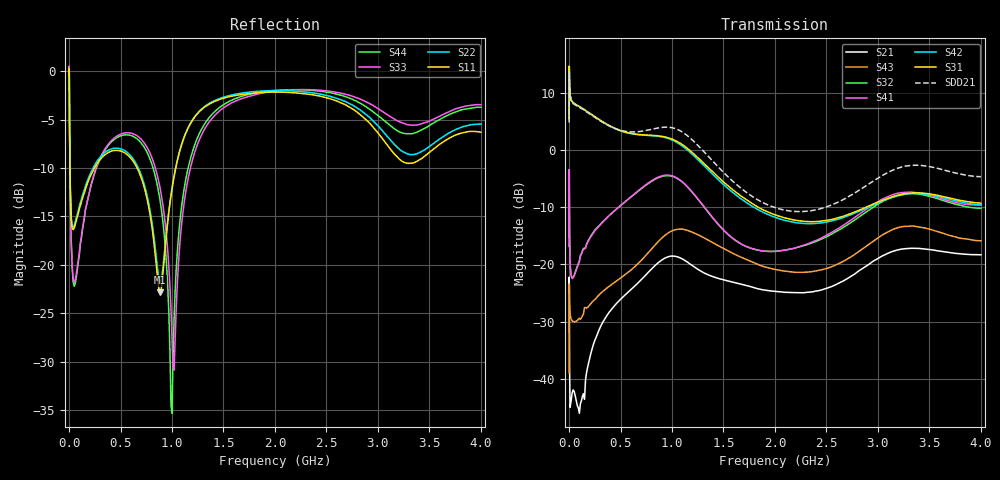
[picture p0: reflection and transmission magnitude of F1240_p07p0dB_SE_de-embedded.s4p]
! Integrated Device Technology
! Corporate Headquarters
! 6024 Silver Creek Valley Road
! San Jose, CA 95138  USA
! Phone:  1-408-284-8200
! Toll Free:  1-800-223-1366
! Webpage:  http://www.idt.com/
! Timing and RF Division
! 515 Groton Road, Suite 102
! Westford, MA 01886-6024
! Device:  F1240
! Description: Dual Intermediate Frequency Digital Variable Gain Amplifier
! Frequency:  10.0 -  500.00 MHz
! Package:  5x5 mm QFN Plastic Package: 32 pin
! Ports:  8 RF, 20 DC
!  Pin  1  = GA3 / Data  Pin 17  = RF OUT_B+
!  Pin  2  = GA4 / CLK  Pin 18  = RF OUT_B-
!  Pin  3  = GA5  Pin 19  = STBY_B
!  Pin  4  = VMODE  Pin 20  = Ground
!  Pin  5  = No Connect  Pin 21  = Ground
!  Pin  6  = GB5  Pin 22  = STB_A
!  Pin  7  = GB4  Pin 23  = RF OUT_A-  = Port 4
!  Pin  8  = GB3  Pin 24  = RF OUT_A+  = Port 3
!  Pin  9  = GB2  Pin 25  = GA0
!  Pin 10  = GB1  Pin 26  = ISET_A
!  Pin 11  = RF IN_B+  Pin 27  = VCC
!  Pin 12  = RF IN_B-  Pin 28  = Ground
!  Pin 13  = Ground  Pin 29  = RF IN_A-  = Port 2
!  Pin 14  = VCC  Pin 30  = RF IN_A+  = Port 1
!  Pin 15  = ISET_B  Pin 31  = GA1
!  Pin 16  = GB0  Pin 32  = GA2 / CSb
! Gain  = +19.5 dB
! State  = 1
! Voltage  = +5.00 V
! Current  = 85.292 mA (one channel only)
! Temperture  =  +25 C
! Test Date  =  2017-10-18
! Board  =  EB4031
! Data:  The device was measured on a custom evaluation board which has
!  individual transmission lines to the RF pins.  Data was collected
!  using a calibrated network analyzer.  The evaluation board was
!  de-embedded using Automatic Fixture Removal.
!  The reference plane is the edge of the package pin.
!  Only Channel A was measured.
!  This data is in single-ended operation.  If your needs are balanced
!  or differential S-parameters then this file needs to be used a
!  linear simulator.
! File Date:  2017-11-10  MJV
! Note:
!  Integrated Device Technology supplies this data as a sample of measured
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# Hz S dB R 100
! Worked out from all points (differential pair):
!   410 points, 500 kHz to 4 GHz, reference 100 ohm
!   strongest paths, dB at 500 kHz, 930 MHz, 1.96 GHz, 2.98 GHz, 4 GHz:
!     S31: 5.6, 2.4, -11.0, -9.2, -9.2
!     S42: 5.5, 2.2, -11.5, -9.4, -9.5
!     S41: -16.7, -4.4, -17.7, -9.2, -9.5
!     S32: -16.9, -4.5, -17.7, -9.7, -10.2
!     S43: -39.0, -14.9, -20.7, -15.6, -15.9
!     S21: -25.0, -18.9, -24.6, -19.2, -18.3
!   taken as a pair (ports 1,2 in; 3,4 out), SDD21 dB: 4.9, 4.1, -9.8, -5.1, -4.6
!   lowest |S11| = -22.8 dB at 880 MHz (marker M1), VSWR 1.16, Z = 111 + j10.7 ohm
!   |S11| at or under -10 dB: 8.743 MHz to 246.3 MHz (237.6 MHz wide, 186 % of centre); 661.2 MHz to 1.036 GHz (374.8 MHz wide, 44.2 % of centre)
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500000  -0.43 -5.5  -25.02 -6.0  -27.16 83.0  -57.48 70.7
        -25.00 -6.1  -0.43 -5.5  -57.70 72.0  -27.16 84.1
        5.57 -105.0  -16.87 -96.5  -0.51 1.5  -39.05 -86.1
        -16.72 -95.8  5.54 -103.9  -38.96 -85.7  -0.52 3.8
3000000  -2.38 -59.6  -27.90 -106.1  -15.26 28.3  -47.33 -69.5
         -27.98 -105.9  -2.34 -59.6  -47.16 -69.5  -15.27 28.4
         13.97 178.7  -7.17 153.0  -1.84 -54.9  -24.04 -164.6
         -7.26 152.8  13.97 178.9  -23.99 -164.6  -1.90 -54.7
3e7  -16.19 -116.0  -42.28 2.6  -15.36 -7.6  -48.21 102.3
     -42.48 1.7  -16.00 -116.1  -48.05 102.5  -15.34 -7.5
     8.53 162.3  -22.32 119.3  -20.05 -104.7  -30.02 162.9
     -22.48 119.8  8.56 162.4  -29.87 162.9  -20.34 -104.8
1.9e8  -11.26 -141.5  -37.59 56.7  -16.79 -48.0  -34.36 31.2
       -37.22 56.9  -10.99 -142.2  -34.33 31.9  -16.80 -48.1
       6.62 112.9  -15.66 33.8  -12.77 -107.0  -27.59 105.6
       -15.79 33.9  6.61 112.3  -27.33 105.1  -12.85 -105.8
8.8e8  -22.83 41.8  -19.75 -86.2  -15.95 172.7  -26.14 -135.8
       -19.49 -90.6  -21.74 43.4  -26.35 -128.7  -16.20 172.1
       2.51 -62.1  -4.72 -165.5  -11.85 135.3  -16.41 -68.6
       -4.61 -168.8  2.43 -63.7  -15.74 -70.3  -13.09 135.3
1.2e9  -5.05 -112.1  -19.70 -178.0  -18.18 83.8  -25.24 150.0
       -20.24 178.2  -4.99 -111.6  -24.77 156.9  -18.77 82.6
       -0.44 -156.1  -7.44 81.2  -9.11 -97.7  -14.83 -168.5
       -7.39 76.4  -0.75 -157.9  -14.37 -170.5  -8.26 -102.2
4e9  -6.29 -149.7  -18.40 86.8  -20.21 -68.7  -21.50 -48.4
     -18.30 86.3  -5.46 -147.6  -22.45 -28.6  -21.70 -61.3
     -9.25 25.9  -10.17 -89.4  -3.45 -140.0  -17.18 80.9
     -9.55 -104.1  -9.53 33.3  -15.85 58.4  -3.71 -147.8
